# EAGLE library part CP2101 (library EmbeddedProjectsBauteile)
Single-Chip USB to UART Bridge Source: www.silabs.com .. CP2101.pdf / cp2102.pdf
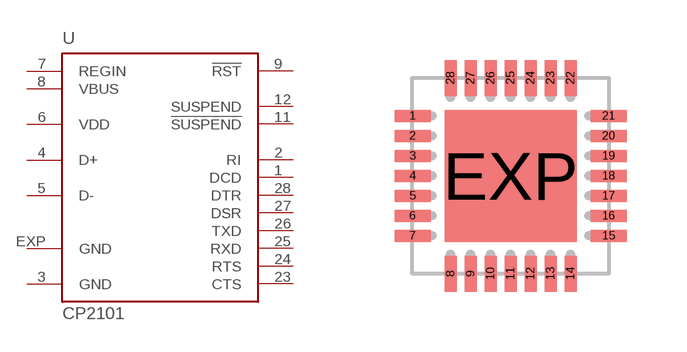
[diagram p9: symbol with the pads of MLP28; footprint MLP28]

Designator prefix -

## CP2101 (EP: 400135)  [MLP28]
1  DCD  in
2  RI  in
3  GND  pwr
4  D+
5  D-
6  VDD  pwr
7  REGIN  pas
8  VBUS  in
9  !RST
11  !SUSPEND  out
12  SUSPEND  out
23  CTS  in
24  RTS  out
25  RXD  in
26  TXD  out
27  DSR  in
28  DTR  out
EXP  GND

## Footprint MLP28 (pad centres in mm)
smd 0.9 x 0.3: 1 -4.99,1.5; 2 -4.99,1; 3 -4.99,0.5; 4 -4.99,0; 5 -4.99,-0.5; 6 -4.99,-1; 7 -4.99,-1.5; 15 -0.09,-1.5; 16 -0.09,-1; 17 -0.09,-0.5; 18 -0.09,0; 19 -0.09,0.5; 20 -0.09,1; 21 -0.09,1.5
smd 0.3 x 0.9: 8 -4.04,-2.45; 9 -3.54,-2.45; 10 -3.04,-2.45; 11 -2.54,-2.45; 12 -2.04,-2.45; 13 -1.54,-2.45; 14 -1.04,-2.45; 22 -1.04,2.45; 23 -1.54,2.45; 24 -2.04,2.45; 25 -2.54,2.45; 26 -3.04,2.45; 27 -3.54,2.45; 28 -4.04,2.45
smd 3.3 x 3.3: EXP -2.54,0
